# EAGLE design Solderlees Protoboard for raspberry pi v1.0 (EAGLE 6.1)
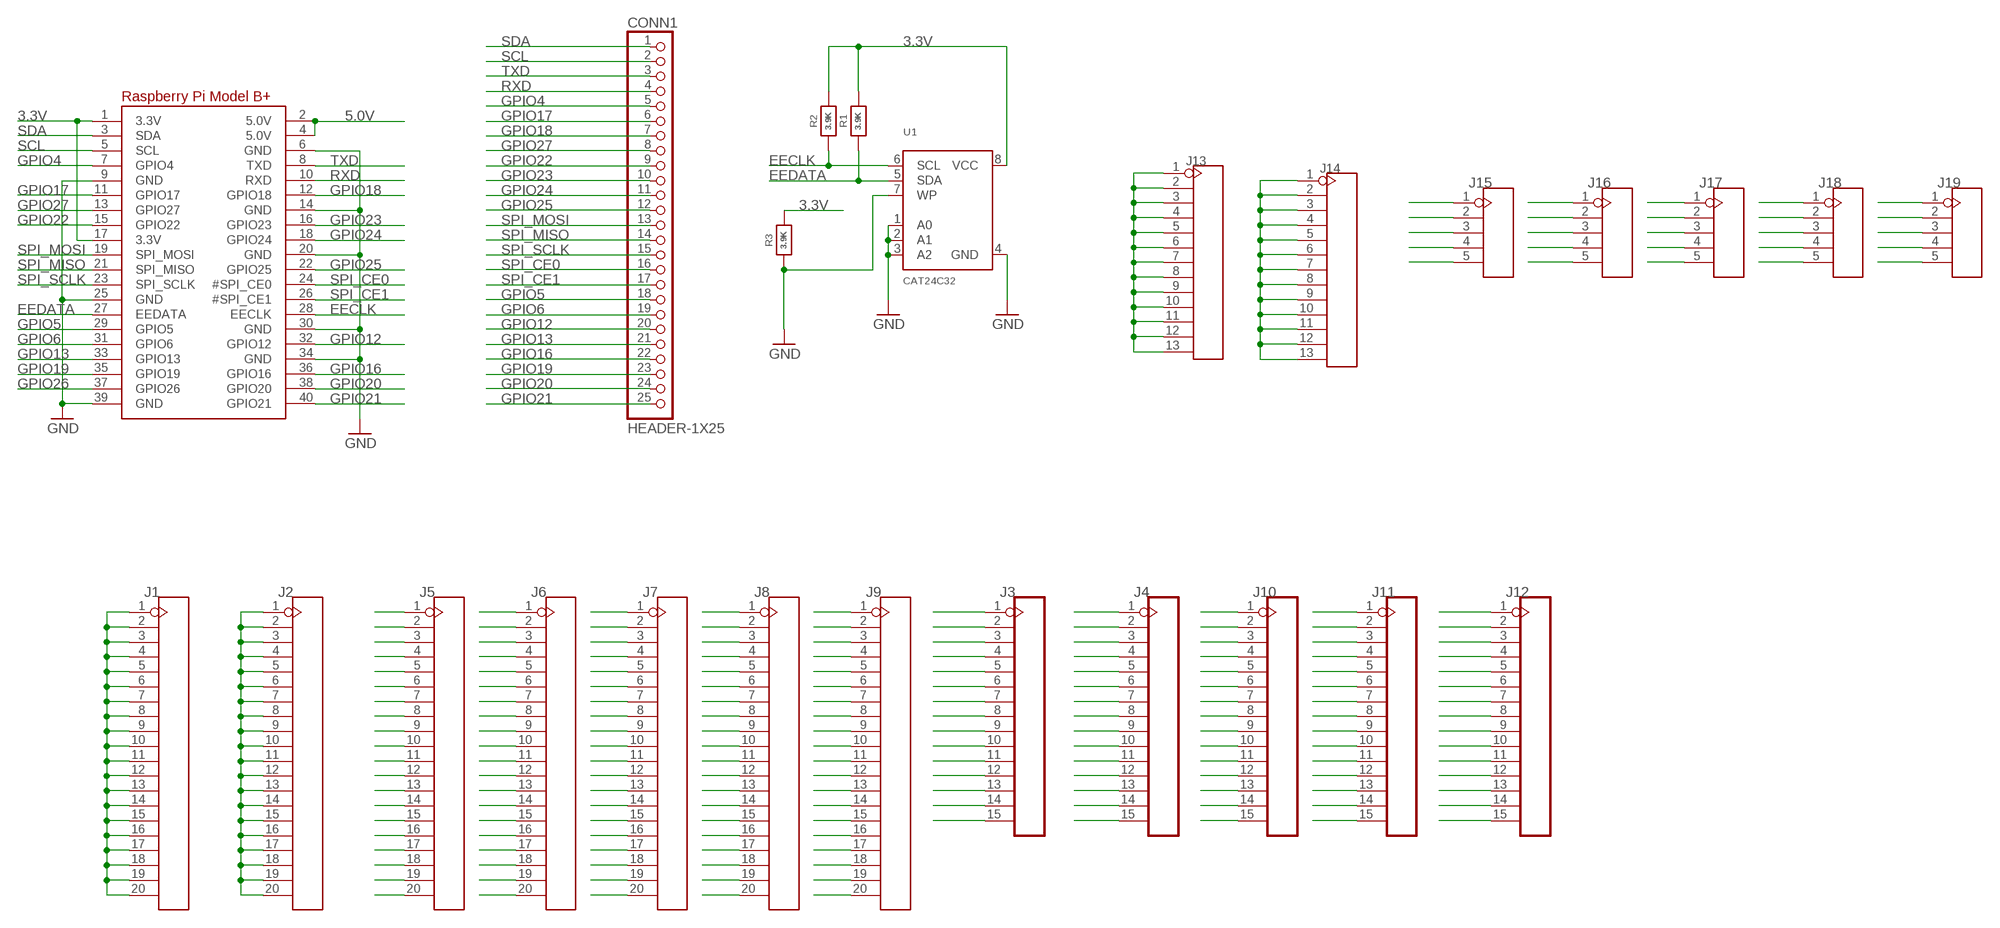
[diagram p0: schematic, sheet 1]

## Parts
CONN1  HEADER-1X25  [1X25_ROUND_70MIL]
J1  HEADER-20P-2.54  [20P-2.54]
J2  HEADER-20P-2.54  [20P-2.54]
J3  HEADER-15P'2.54'  [15P-2.54]
J4  HEADER-15P'2.54'  [15P-2.54]
J5  HEADER-20P-2.54  [20P-2.54]
J6  HEADER-20P-2.54  [20P-2.54]
J7  HEADER-20P-2.54  [20P-2.54]
J8  HEADER-20P-2.54  [20P-2.54]
J9  HEADER-20P-2.54  [20P-2.54]
J10  HEADER-15P'2.54'  [15P-2.54]
J11  HEADER-15P'2.54'  [15P-2.54]
J12  HEADER-15P'2.54'  [15P-2.54]
J13  HEADER-13P  [13P-2.54]
J14  HEADER-13P  [13P-2.54]
J15  HEADER-5P-2.54  [5P-2.54]
J16  HEADER-5P-2.54  [5P-2.54]
J17  HEADER-5P-2.54  [5P-2.54]
J18  HEADER-5P-2.54  [5P-2.54]
J19  HEADER-5P-2.54  [5P-2.54]
R1  3.9K  RESISTOR0805_NOOUTLINE  [0805-NO]
R2  3.9K  RESISTOR0805_NOOUTLINE  [0805-NO]
R3  3.9K  RESISTOR0805_NOOUTLINE  [0805-NO]
RPI1  RASPBERRYPI_BPLUS_HATNOSLOTS  [PI_HAT_NOSLOTS]
U1  CAT24C32  EEPROM_I2C_SOIC8_GENERIC  [SOIC8_150MIL]

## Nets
1: J5.1 J6.1 J7.1 J8.1 J9.1
01: J15.1 J16.1 J17.1 J18.1 J19.1
2: J5.2 J6.2 J7.2 J8.2 J9.2
02: J15.2 J16.2 J17.2 J18.2 J19.2
3: J5.3 J6.3 J7.3 J8.3 J9.3
03: J15.3 J16.3 J17.3 J18.3 J19.3
3.3V: J1.1 J1.2 J1.3 J1.4 J1.5 J1.6 J1.7 J1.8 J1.9 J1.10 J1.11 J1.12 J1.13 J1.14 J1.15 J1.16 J1.17 J1.18 J1.19 J1.20 R1.2 R2.2 R3.2 RPI1.1(3.3V) RPI1.17(3.3V) U1.8(VCC)
4: J5.4 J6.4 J7.4 J8.4 J9.4
04: J15.4 J16.4 J17.4 J18.4 J19.4
5: J5.5 J6.5 J7.5 J8.5 J9.5
05: J15.5 J16.5 J17.5 J18.5 J19.5
5.0V: J13.1 J13.2 J13.3 J13.4 J13.5 J13.6 J13.7 J13.8 J13.9 J13.10 J13.11 J13.12 J13.13 RPI1.2(5.0V) RPI1.4(5.0V)
6: J5.6 J6.6 J7.6 J8.6 J9.6
7: J5.7 J6.7 J7.7 J8.7 J9.7
8: J5.8 J6.8 J7.8 J8.8 J9.8
9: J5.9 J6.9 J7.9 J8.9 J9.9
10: J5.10 J6.10 J7.10 J8.10 J9.10
11: J5.11 J6.11 J7.11 J8.11 J9.11
12: J5.12 J6.12 J7.12 J8.12 J9.12
13: J5.13 J6.13 J7.13 J8.13 J9.13
14: J5.14 J6.14 J7.14 J8.14 J9.14
15: J5.15 J6.15 J7.15 J8.15 J9.15
16: J5.16 J6.16 J7.16 J8.16 J9.16
17: J5.17 J6.17 J7.17 J8.17 J9.17
18: J5.18 J6.18 J7.18 J8.18 J9.18
19: J5.19 J6.19 J7.19 J8.19 J9.19
20: J5.20 J6.20 J7.20 J8.20 J9.20
22: J3.2 J4.2 J10.2 J11.2 J12.2
33: J3.3 J4.3 J10.3 J11.3 J12.3
44: J3.4 J4.4 J10.4 J11.4 J12.4
55: J3.5 J4.5 J10.5 J11.5 J12.5
66: J3.6 J4.6 J10.6 J11.6 J12.6
77: J3.7 J4.7 J10.7 J11.7 J12.7
88: J3.8 J4.8 J10.8 J11.8 J12.8
99: J3.9 J4.9 J10.9 J11.9 J12.9
100: J3.10 J4.10 J10.10 J11.10 J12.10
101: J3.11 J4.11 J10.11 J11.11 J12.11
102: J3.12 J4.12 J10.12 J11.12 J12.12
103: J3.13 J4.13 J10.13 J11.13 J12.13
104: J3.14 J4.14 J10.14 J11.14 J12.14
105: J3.15 J4.15 J10.15 J11.15 J12.15
111: J3.1 J4.1 J10.1 J11.1 J12.1
EECLK: R2.1 RPI1.28(EECLK) U1.6(SCL)
EEDATA: R1.1 RPI1.27(EEDATA) U1.5(SDA)
GND: J2.1 J2.2 J2.3 J2.4 J2.5 J2.6 J2.7 J2.8 J2.9 J2.10 J2.11 J2.12 J2.13 J2.14 J2.15 J2.16 J2.17 J2.18 J2.19 J2.20 J14.1 J14.2 J14.3 J14.4 J14.5 J14.6 J14.7 J14.8 J14.9 J14.10 J14.11 J14.12 J14.13 R3.1 RPI1.6(GND) RPI1.9(GND) RPI1.14(GND) RPI1.20(GND) RPI1.25(GND) RPI1.30(GND) RPI1.34(GND) RPI1.39(GND) U1.1(A0) U1.2(A1) U1.3(A2) U1.4(GND) U1.7(WP)
GPIO4: CONN1.5 RPI1.7(GPIO4)
GPIO5: CONN1.18 RPI1.29(GPIO5)
GPIO6: CONN1.19 RPI1.31(GPIO6)
GPIO12: CONN1.20 RPI1.32(GPIO12)
GPIO13: CONN1.21 RPI1.33(GPIO13)
GPIO16: CONN1.22 RPI1.36(GPIO16)
GPIO17: CONN1.6 RPI1.11(GPIO17)
GPIO18: CONN1.7 RPI1.12(GPIO18)
GPIO19: CONN1.23 RPI1.35(GPIO19)
GPIO20: CONN1.24 RPI1.38(GPIO20)
GPIO21: CONN1.25 RPI1.40(GPIO21)
GPIO22: CONN1.9 RPI1.15(GPIO22)
GPIO23: CONN1.10 RPI1.16(GPIO23)
GPIO24: CONN1.11 RPI1.18(GPIO24)
GPIO25: CONN1.12 RPI1.22(GPIO25)
GPIO26: RPI1.37(GPIO26)
GPIO27: CONN1.8 RPI1.13(GPIO27)
RXD: CONN1.4 RPI1.10(RXD)
SCL: CONN1.2 RPI1.5(SCL)
SDA: CONN1.1 RPI1.3(SDA)
SPI_CE0: CONN1.16 RPI1.24(#SPI_CE0)
SPI_CE1: CONN1.17 RPI1.26(#SPI_CE1)
SPI_MISO: CONN1.14 RPI1.21(SPI_MISO)
SPI_MOSI: CONN1.13 RPI1.19(SPI_MOSI)
SPI_SCLK: CONN1.15 RPI1.23(SPI_SCLK)
TXD: CONN1.3 RPI1.8(TXD)

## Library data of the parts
CONN1 = microbuilder:HEADER-1X25
J1 J2 J5-J9 = Connector:HEADER-20P
J3 J4 J10-J12 = Connector:HEADER-15P: Header 15 Standard 15-pin 0.1" header. Use with straight break away headers (SKU : PRT-00116), right angle break away headers (PRT-00553), swiss pins (PRT-00743), machine pins (PRT-00117), and female headers (PRT-00115).
J13 J14 = Connector:HEADER-13P
J15-J19 = Connector:HEADER-5P
R1-R3 = microbuilder:RESISTOR: Resistors
RPI1 = microbuilder:RASPBERRYPI_BPLUS
U1 = microbuilder:EEPROM_I2C_SOIC8_GENERIC: Note: The same pinout is used for many I2C EEPROMs in SOIC8(150mil) from a variety of manufacturers and in various sizes. Examples: 16K (2K x 8 Bit) I2C EEPROM 1.7-5.5V, 400KHz, -40°C-85°C Digikey: CAT24C16WI-GT3CT-ND 256K (32K x 8 Bit) I2C EEPROM 1.7-5.5V, 400KHz, -40°C-85°C Digikey: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

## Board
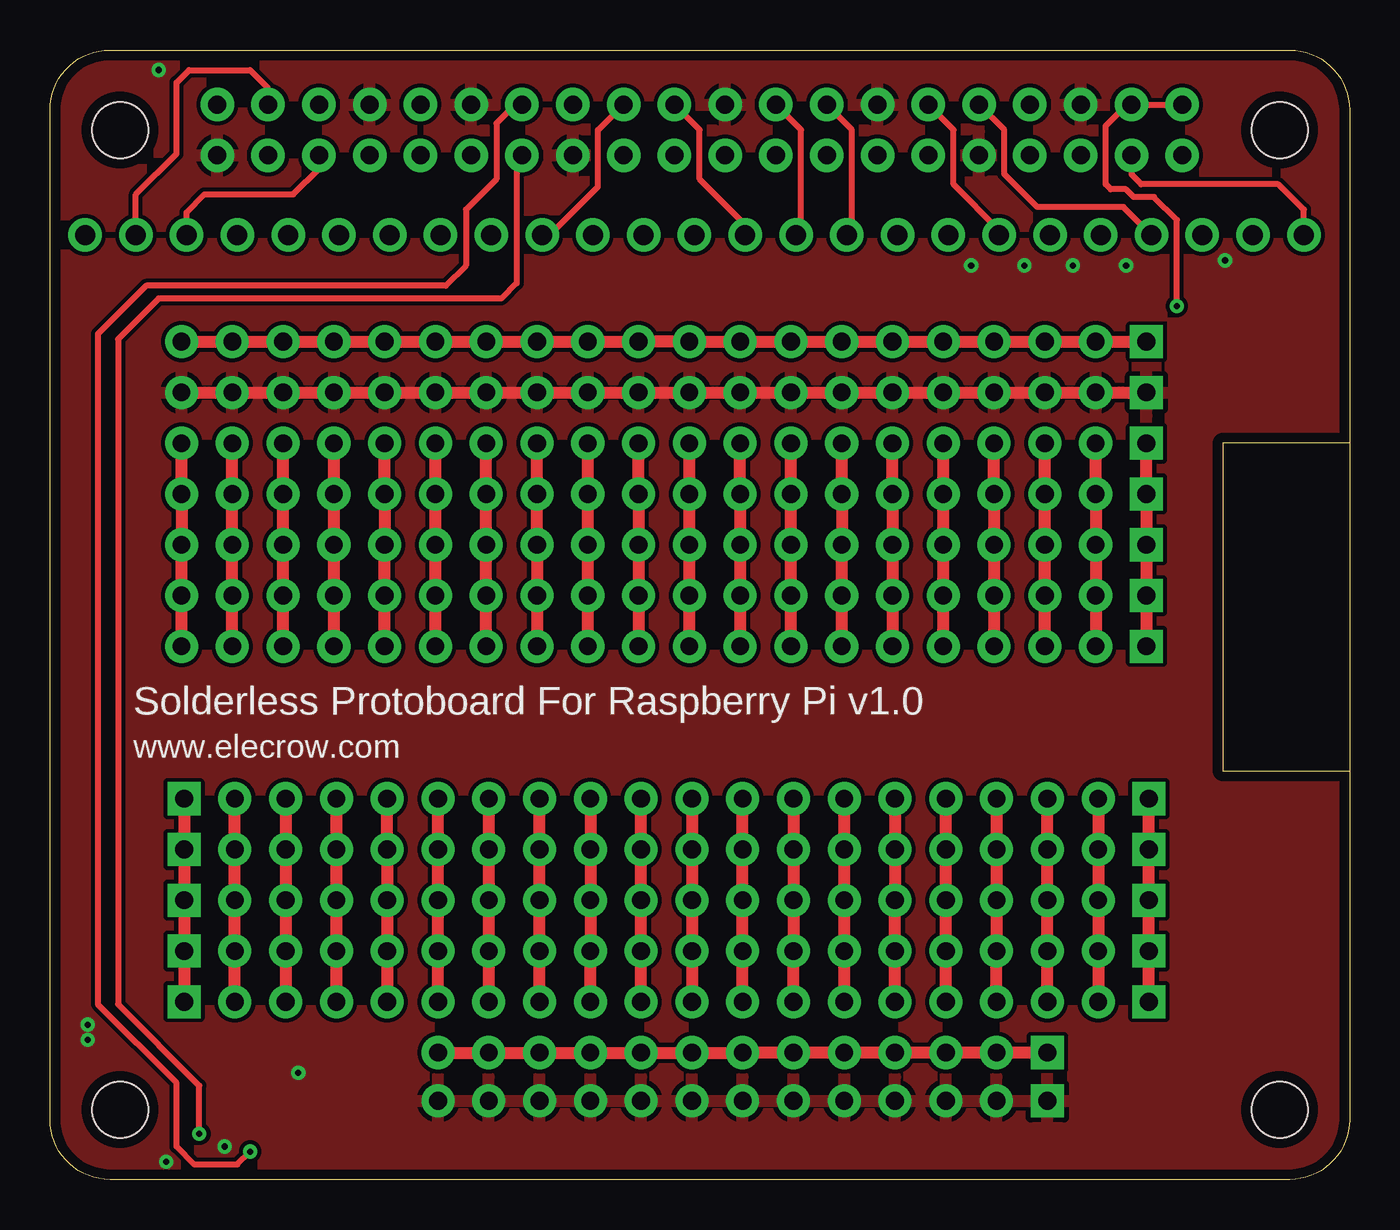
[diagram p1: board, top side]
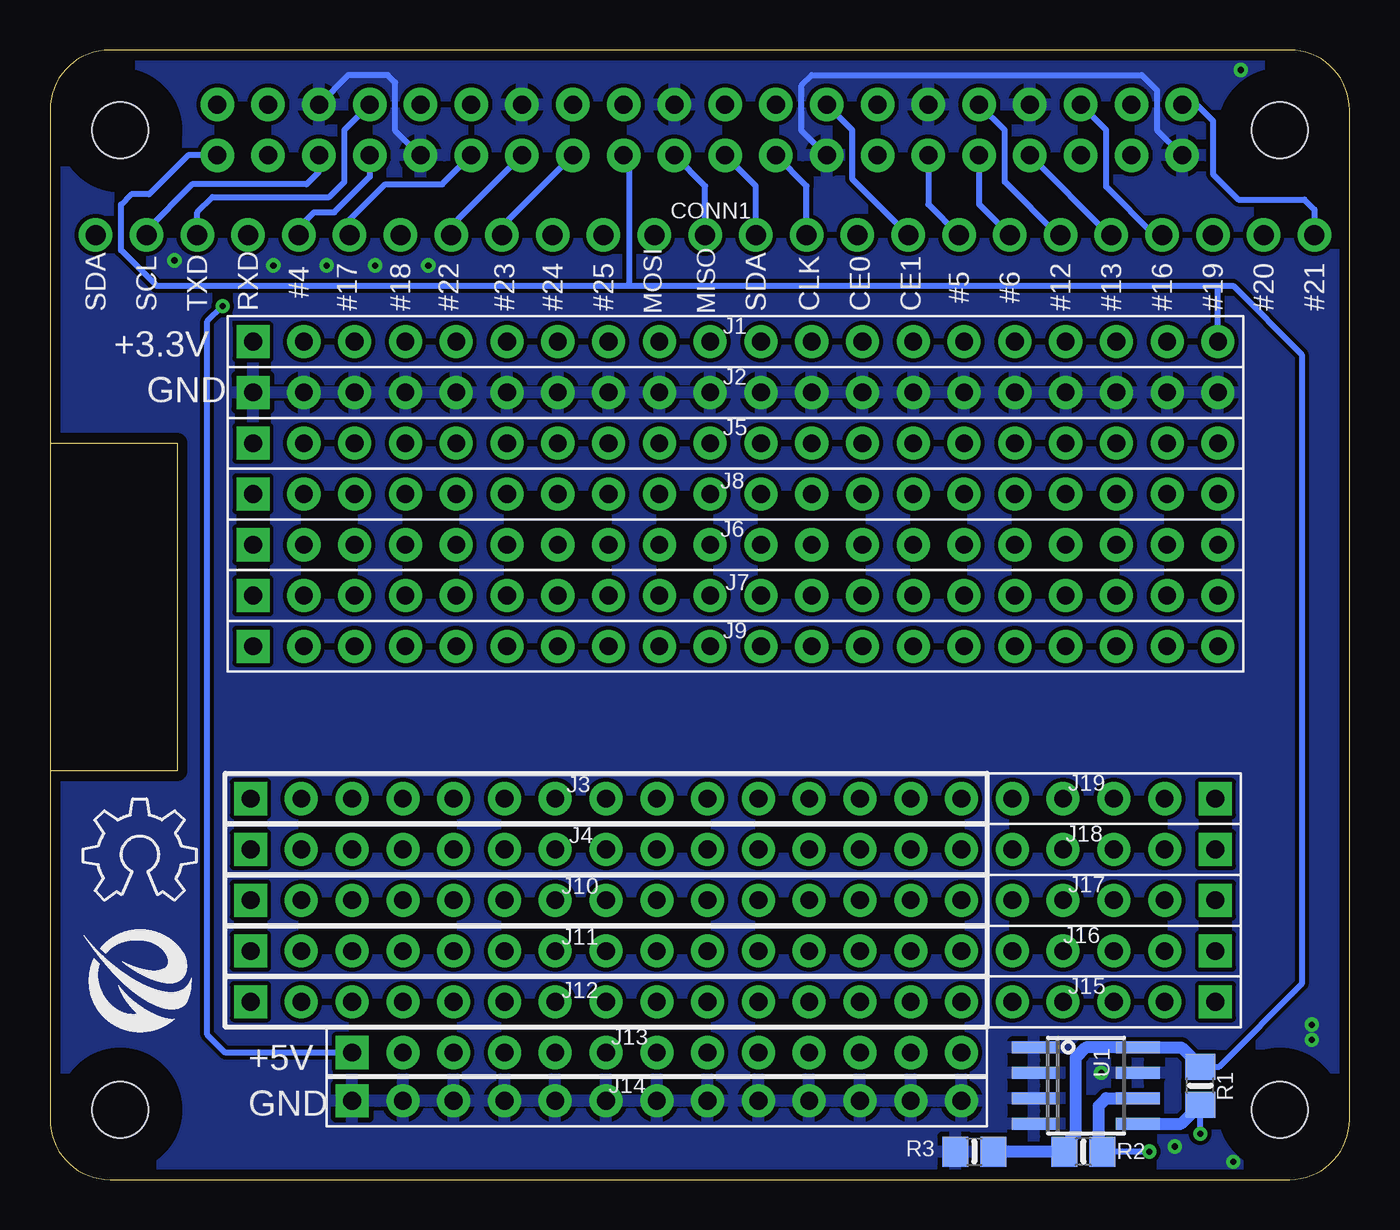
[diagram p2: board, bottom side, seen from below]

Size 65 x 56.5 mm. Coordinates in mm from the lower left corner, seen from the top.
Outline: 65,36.83 58.65,36.83 58.65,20.45 65,20.45
Copper layers (1*16): Top 0.035mm / dielectric 1.5mm / Bottom 0.035mm
Design rules: minimum track width 10mil, minimum drill 10mil, track to track 8mil, track to pad 8mil, pad to pad 8mil, via to via 8mil, smd to smd 8mil, copper to edge 20mil, drill to drill 8mil, minimum pad ring 10mil, minimum via ring 8mil, stop-mask expansion 4mil, vias tented up to drill 100mil, thermal gap 10mil

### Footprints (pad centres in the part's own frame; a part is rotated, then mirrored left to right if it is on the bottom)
1X25_ROUND_70MIL = drill 1 pad 1.676: 1 -30.48,0; 2 -27.94,0; 3 -25.4,0; 4 -22.86,0; 5 -20.32,0; 6 -17.78,0; 7 -15.24,0; 8 -12.7,0; 9 -10.16,0; 10 -7.62,0; 11 -5.08,0; 12 -2.54,0; 13 0,0; 14 2.54,0; 15 5.08,0; 16 7.62,0; 17 10.16,0; 18 12.7,0; 19 15.24,0; 20 17.78,0; 21 20.32,0; 22 22.86,0; 23 25.4,0; 24 27.94,0; 25 30.48,0
20P-2.54 = drill 0.889 pad 1.651 square: 1 -25.4,0 | drill 0.889 pad 1.651: 2 -22.86,0; 3 -20.32,0; 4 -17.78,0; 5 -15.24,0; 6 -12.7,0; 7 -10.16,0; 8 -7.62,0; 9 -5.08,0; 10 -2.54,0; 11 0,0; 12 2.54,0; 13 5.08,0; 14 7.62,0; 15 10.16,0; 16 12.7,0; 17 15.24,0; 18 17.78,0; 19 20.32,0; 20 22.86,0
15P-2.54 = drill 0.889 pad 1.651 square: 1 -17.78,0 | drill 0.889 pad 1.651: 2 -15.24,0; 3 -12.7,0; 4 -10.16,0; 5 -7.62,0; 6 -5.08,0; 7 -2.54,0; 8 0,0; 9 2.54,0; 10 5.08,0; 11 7.62,0; 12 10.16,0; 13 12.7,0; 14 15.24,0; 15 17.78,0
13P-2.54 = drill 0.889 pad 1.651 square: 1 -15.24,0 | drill 0.889 pad 1.651: 2 -12.7,0; 3 -10.16,0; 4 -7.62,0; 5 -5.08,0; 6 -2.54,0; 7 0,0; 8 2.54,0; 9 5.08,0; 10 7.62,0; 11 10.16,0; 12 12.7,0; 13 15.24,0
5P-2.54 = drill 0.889 pad 1.651 square: 1 0,5.08 | drill 0.889 pad 1.651: 2 0,2.54; 3 0,0; 4 0,-2.54; 5 0,-5.08
0805-NO = smd 1.3 x 1.5: 1 -0.95,0; 2 0.95,0
PI_HAT_NOSLOTS = drill 0.9 pad 1.676: 1 8.37,51.23; 2 8.37,53.77; 3 10.91,51.23; 4 10.91,53.77; 5 13.45,51.23; 6 13.45,53.77; 7 15.99,51.23; 8 15.99,53.77; 9 18.53,51.23; 10 18.53,53.77; 11 21.07,51.23; 12 21.07,53.77; 13 23.61,51.23; 14 23.61,53.77; 15 26.15,51.23; 16 26.15,53.77; 17 28.69,51.23; 18 28.69,53.77; 19 31.23,51.23; 20 31.23,53.77; 21 33.77,51.23; 22 33.77,53.77; 23 36.31,51.23; 24 36.31,53.77; 25 38.85,51.23; 26 38.85,53.77; 27 41.39,51.23; 28 41.39,53.77; 29 43.93,51.23; 30 43.93,53.77; 31 46.47,51.23; 32 46.47,53.77; 33 49.01,51.23; 34 49.01,53.77; 35 51.55,51.23; 36 51.55,53.77; 37 54.09,51.23; 38 54.09,53.77; 39 56.63,51.23; 40 56.63,53.77 | hole 2.8: 3.5,3.5; 3.5,52.5; 61.5,52.5; 61.5,3.5
SOIC8_150MIL = smd 0.6 x 2.2: 1 -1.905,-2.6; 2 -0.635,-2.6; 3 0.635,-2.6; 4 1.905,-2.6; 5 1.905,2.6; 6 0.635,2.6; 7 -0.635,2.6; 8 -1.905,2.6

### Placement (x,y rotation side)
CONN1  32.23,47.24 0 bottom
J1  29.44,41.91 0 bottom
J2  29.44,39.37 0 bottom
J3  37.19,19.05 0 bottom
J4  37.19,16.51 0 bottom
J5  29.44,36.83 0 bottom
J6  29.44,31.75 0 bottom
J7  29.44,29.21 0 bottom
J8  29.44,34.29 0 bottom
J9  29.44,26.67 0 bottom
J10  37.19,13.97 0 bottom
J11  37.19,11.43 0 bottom
J12  37.19,8.89 0 bottom
J13  34.65,6.35 0 bottom
J14  34.65,3.94 0 bottom
J15  11.79,8.89 270 bottom
J16  11.79,11.43 270 bottom
J17  11.79,13.97 270 bottom
J18  11.79,16.51 270 bottom
J19  11.79,19.05 270 bottom
R1  7.47,4.7 90 bottom
R2  13.31,1.4 180 bottom
R3  18.77,1.4 0 bottom
RPI1  65,0 0 bottom
U1  13.18,4.7 270 bottom
U$1  [ELECROW-NEW]  63.35,7.37 0 bottom
U$2  [OSHW_6X200_NOTEXT]  63.35,13.97 0 bottom

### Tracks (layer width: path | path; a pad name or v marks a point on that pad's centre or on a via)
1
  Top 0.61: J5.1 J8.1 J6.1 J7.1 J9.1
01
  Top 0.61: J19.1 J18.1 J17.1 J16.1 J15.1
2
  Top 0.61: J5.2 J8.2 J6.2 J7.2 J9.2
02
  Top 0.61: J15.2 J16.2 J17.2 J18.2 J19.2
3
  Top 0.61: J5.3 J8.3 J6.3 J7.3 J9.3
03
  Top 0.61: J19.3 J18.3 J17.3 J16.3 J15.3
3.3V
  Top 0.61: J1.1 J1.2 J1.3 J1.4 J1.5 J1.6 J1.7 J1.8 J1.9 J1.10 J1.11 J1.12 J1.13 J1.14 J1.15 J1.16 J1.17 J1.18 J1.19 J1.20
  Bottom 0.305: RPI1.17 36.31,50.81 36.04,50.55 36.04,44.7 | 36.04,44.7 59.67,44.7 61.44,46.48 61.44,48.77 60.94,49.28 60.05,49.28 58.09,51.23 RPI1.1 | 36.04,44.7 6.58,44.7 | 6.58,44.7 5.82,44.7 2.39,41.27 2.39,9.78 6.52,5.65 R1.2 | J1.20 6.58,44.7
  Bottom 0.61: R3.2 R2.2 14.2,1.4 14.2,1.78 13.69,2.29 13.69,6.1 13.18,6.6 U1.8 8.42,6.6 R1.2
4
  Top 0.61: J5.4 J8.4 J6.4 J7.4 J9.4
04
  Top 0.61: J15.4 J16.4 J17.4 J18.4 J19.4
5
  Top 0.61: J5.5 J8.5 J6.5 J7.5 J9.5
05
  Top 0.61: J19.5 J18.5 J17.5 J16.5 J15.5
5.0V  (via drill 0.3)
  Top 0.305: RPI1.2 RPI1.4 53.87,53.77 52.81,52.7 52.81,49.78 53.06,49.53 53.82,49.53 54.2,49.15 55.22,49.15 56.36,48.01 v56.36,43.69
  Top 0.61: J13.13 J13.12 J13.11 J13.10 J13.9 J13.8 J13.7 J13.6 J13.5 J13.4 J13.3 J13.2 J13.1
  Bottom 0.305: J13.1 56.24,6.35 57.13,7.24 57.13,42.93 v56.36,43.69
6
  Top 0.61: J5.6 J8.6 J6.6 J7.6 J9.6
7
  Top 0.61: J5.7 J8.7 J6.7 J7.7 J9.7
8
  Top 0.61: J9.8 J7.8 J6.8 J8.8 J5.8
9
  Top 0.61: J5.9 J8.9 J6.9 J7.9 J9.9
10
  Top 0.61: J9.10 J7.10 J6.10 J8.10 J5.10
11
  Top 0.61: J5.11 J8.11 J6.11 J7.11 J9.11
12
  Top 0.61: J5.12 J8.12 J6.12 J7.12 J9.12
13
  Top 0.61: J5.13 J8.13 J6.13 J7.13 J9.13
14
  Top 0.61: J5.14 J8.14 J6.14 J7.14 J9.14
15
  Top 0.61: J5.15 J8.15 J6.15 J7.15 J9.15
16
  Top 0.61: J5.16 J8.16 J6.16 J7.16 J9.16
17
  Top 0.61: J9.17 J7.17 J6.17 J8.17 J5.17
18
  Top 0.61: J5.18 J8.18 J6.18 J7.18 J9.18
19
  Top 0.61: J9.19 J7.19 J6.19 J8.19 J5.19
20
  Top 0.61: J5.20 J8.20 J6.20 J7.20 J9.20
22
  Top 0.61: J3.2 J4.2 J10.2 J11.2 J12.2
33
  Top 0.61: J12.3 J11.3 J10.3 J4.3 J3.3
44
  Top 0.61: J3.4 J4.4 J10.4 J11.4 J12.4
55
  Top 0.61: J12.5 J11.5 J10.5 J4.5 J3.5
66
  Top 0.61: J3.6 J4.6 J10.6 J11.6 J12.6
77
  Top 0.61: J12.7 J11.7 J10.7 J4.7 J3.7
88
  Top 0.61: J3.8 J4.8 J10.8 J11.8 J12.8
99
  Top 0.61: J12.9 J11.9 J10.9 J4.9 J3.9
100
  Top 0.61: J3.10 J4.10 J10.10 J11.10 J12.10
101
  Top 0.61: J12.11 J11.11 J10.11 J4.11 J3.11
102
  Top 0.61: J3.12 J4.12 J10.12 J11.12 J12.12
103
  Top 0.61: J12.13 J11.13 J10.13 J4.13 J3.13
104
  Top 0.61: J3.14 J4.14 J10.14 J11.14 J12.14
105
  Top 0.61: J12.15 J11.15 J10.15 J4.15 J3.15
111
  Top 0.61: J12.1 J11.1 J10.1 J4.1 J3.1
EECLK  (via drill 0.3)
  Top 0.305: RPI1.28 23.27,53.77 22.33,52.83 22.33,50.04 20.8,48.51 20.8,45.72 19.79,44.7 4.8,44.7 2.39,42.29 2.39,8.76 6.33,4.83 6.33,1.65 7.21,0.76 9.37,0.76 v10.01,1.4
  Bottom 0.305: v10.01,1.4 R2.1
  Bottom 0.61: R2.1 12.36,1.72 12.55,1.91 12.55,3.68 12.17,4.06 U1.6
EEDATA  (via drill 0.3)
  Top 0.305: RPI1.27 23.61,51.19 23.34,50.93 23.34,44.83 22.58,44.07 5.44,44.07 3.4,42.04 3.4,8.76 7.47,4.7 v7.47,2.29
  Bottom 0.305: v7.47,2.29 R1.1
  Bottom 0.61: U1.5 8.42,2.79 R1.1
GND  (via drill 0.3)
  Top 0.61: J2.20 J2.19 J2.18 J2.17 J2.16 J2.15 J2.14 J2.13 J2.12 J2.11 J2.10 J2.9 J2.8 J2.7 J2.6 J2.5 J2.4 J2.3 J2.2 J2.1
  Bottom 0.305: RPI1.9 46.51,51.23 47.73,52.45 47.73,54.86 48.11,55.24 50.08,55.24 RPI1.6 | RPI1.25 26.19,51.23 27.41,52.45 27.41,54.74 26.9,55.24 10.39,55.24 9.63,54.48 9.63,52.49 RPI1.39
  other vias: 12.42,5.33 1.88,6.99 1.88,7.75 8.74,1.65 5.82,0.89 58.78,45.97 53.82,45.72 51.16,45.72 48.74,45.72 46.08,45.72 5.44,55.5
  pour Bottom: -1.04,56.77 -1.04,0.13 arc90 0.23,-1.14 65,-1.14 arc90 66.27,0.13 66.27,56.77 arc90 65,58.04 0.23,58.04 arc90
  pour Top: 66.27,0 66.14,0 66.14,56.77 arc90 64.87,58.04 0.23,58.04 arc90 -1.04,56.77 -1.04,0.13 arc90 0.23,-1.14 65.13,-1.14 arc90
GPIO4
  Bottom 0.305: CONN1.5 52.55,47.62 51.79,48.39 50.78,48.39 49.01,50.15 RPI1.7
GPIO5
  Bottom 0.305: RPI1.29 21.07,48.78 CONN1.18
GPIO6
  Bottom 0.305: RPI1.31 18.53,48.78 CONN1.19
GPIO12
  Bottom 0.305: CONN1.20 14.58,47.24 17.25,49.91 17.25,52.49 RPI1.32
GPIO13
  Bottom 0.305: CONN1.21 12,47.24 RPI1.33
GPIO16
  Bottom 0.305: CONN1.22 9.76,47.24 12.17,49.66 12.17,52.49 RPI1.36
GPIO17
  Bottom 0.305: CONN1.6 50.01,48.01 48.24,49.78 45.38,49.78 RPI1.11
GPIO18
  Top 0.305: CONN1.7 47.47,47.5 45.19,49.78 45.19,52.51 RPI1.12
GPIO19
  Top 0.305: CONN1.23 6.83,48.39 7.72,49.28 12.17,49.28 13.45,50.56 RPI1.35
GPIO20
  Top 0.305: CONN1.24 4.29,49.28 6.33,51.31 6.33,54.86 6.96,55.5 10.01,55.5 10.91,54.6 RPI1.38
GPIO21
  Bottom 0.305: CONN1.25 1.75,48.51 2.26,49.02 5.56,49.02 6.83,50.29 6.83,52.96 7.64,53.77 RPI1.40
GPIO22
  Bottom 0.305: CONN1.9 42.39,47.69 RPI1.15
GPIO23
  Top 0.305: RPI1.16 40.11,52.51 40.11,47.5 CONN1.10
GPIO24
  Top 0.305: CONN1.11 37.57,47.5 37.57,52.51 RPI1.18
GPIO25
  Top 0.305: CONN1.12 34.77,47.75 32.49,50.04 32.49,52.51 RPI1.22
GPIO27
  Bottom 0.305: CONN1.8 44.93,47.69 RPI1.13
RXD
  Top 0.305: RPI1.10 47.73,52.51 47.73,50.29 49.38,48.64 53.7,48.64 CONN1.4
SCL
  Bottom 0.305: RPI1.5 51.54,51.22 51.54,50.42 52.17,49.78 57.89,49.78 60.17,47.5 CONN1.2
SDA
  Top 0.305: CONN1.1 62.71,48.51 61.44,49.78 54.59,49.78 54.09,50.28 RPI1.3
SPI_CE0
  Top 0.305: CONN1.16 25,47.24 27.41,49.66 27.41,52.49 RPI1.24
SPI_CE1
  Bottom 0.305: CONN1.17 24.87,50.04 24.87,52.49 RPI1.26
SPI_MISO
  Bottom 0.305: CONN1.14 29.69,49.69 RPI1.21
SPI_MOSI
  Bottom 0.305: CONN1.13 32.23,49.69 RPI1.19
SPI_SCLK
  Bottom 0.305: CONN1.15 27.15,49.69 RPI1.23
TXD
  Bottom 0.305: CONN1.3 57.63,48.39 56.87,49.15 51.03,49.15 50.27,49.91 50.27,52.51 RPI1.8

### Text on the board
tNames: Solderless Protoboard For Raspberry Pi v1.0 | www.elecrow.com
bNames: #6 | #5 | #4 | #21 | #20 | #19 | #16 | #13 | #12 | CE1 | CE0 | CLK | SDA | MISO | MOSI | #25 | #24 | #23 | #22 | #18 | #17 | RXD | TXD | SCL | SDA | +3.3V | GND | +5V | GND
